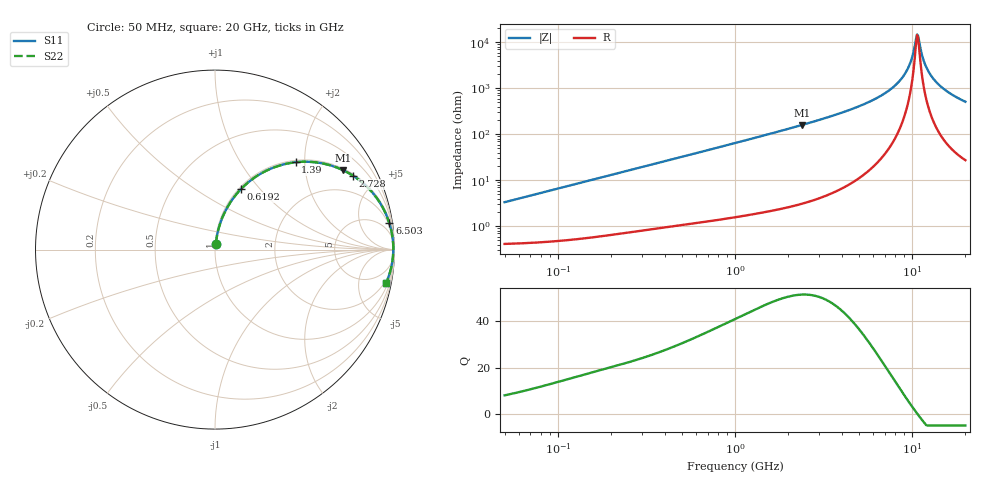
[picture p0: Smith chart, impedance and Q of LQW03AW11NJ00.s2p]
!Murata Part Number: LQW03AW11NJ00
!These Parameters are Measured in Series Mode Connection
!  o--[Z]--o
!Port1  Port2
!  o-------o
!Freq. Start=50[MHz] Stop=20[GHz], 401[Steps]
# Hz S RI R 50
!Freq.(Hz) S11(Real) S11(Imag) S21(Real) S21(Imag) S12(Real) S12(Imag) S22(Real) S22(Imag)
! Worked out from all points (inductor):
!   401 points, 50 MHz to 20 GHz, reference 50 ohm
!   read as one part in series: L = 10.6 nH near 51.52 MHz
!   highest Q = 51.5 at 2.384 GHz (marker M1), where L = 10.6 nH
!   self-resonance near 10.66 GHz
!   S11 on the Smith chart (normalised r, x): 50 MHz: 1.01, +0.07; 619.2 MHz: 1.02, +0.80; 1.39 GHz: 1.04, +1.80; 2.728 GHz: 1.07, +3.70; 6.503 GHz: 2, +13; 20 GHz: 2, -10
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5e7  0.00522 0.0329  0.9948 -0.0329  0.9948 -0.0329  0.00522 0.0329
1.364002e8  0.0133 0.0883  0.9867 -0.0883  0.9867 -0.0883  0.0133 0.0883
3.721004e8  0.0626 0.2243  0.9374 -0.2243  0.9374 -0.2243  0.0626 0.2243
6.192061e8  0.145 0.3375  0.855 -0.3375  0.855 -0.3375  0.145 0.3375
1e9  0.2983 0.4455  0.7017 -0.4455  0.7017 -0.4455  0.2983 0.4455
1.390315e9  0.4493 0.4867  0.5507 -0.4867  0.5507 -0.4867  0.4493 0.4867
2.383959e9  0.7135 0.4425  0.2865 -0.4425  0.2865 -0.4425  0.7135 0.4425
2.728004e9  0.7697 0.4114  0.2303 -0.4114  0.2303 -0.4114  0.7697 0.4114
4.472136e9  0.9163 0.265  0.0837 -0.265  0.0837 -0.265  0.9163 0.265
6.503449e9  0.9713 0.1479  0.0287 -0.1479  0.0287 -0.1479  0.9713 0.1479
7.442007e9  0.9822 0.1071  0.0178 -0.1071  0.0178 -0.1071  0.9822 0.1071
8.516016e9  0.9893 0.0671  0.0107 -0.0671  0.0107 -0.0671  0.9893 0.0671
9.316812e9  0.992 0.0407  0.00796 -0.0407  0.00796 -0.0407  0.992 0.0407
9.892087e9  0.9931 0.0232  0.00693 -0.0232  0.00693 -0.0232  0.9931 0.0232
1.050288e10  0.9935 0.00581  0.00655 -0.00581  0.00655 -0.00581  0.9935 0.00581
1.066139e10  0.9934 0.00146  0.00655 -0.00146  0.00655 -0.00146  0.9934 0.00146
1.098561e10  0.9933 -0.00725  0.00668 0.00725  0.00668 0.00725  0.9933 -0.00725
1.149051e10  0.9928 -0.0203  0.00718 0.0203  0.00718 0.0203  0.9928 -0.0203
1.201863e10  0.992 -0.0334  0.00804 0.0334  0.00804 0.0334  0.992 -0.0334
1.314879e10  0.9891 -0.0596  0.0109 0.0596  0.0109 0.0596  0.9891 -0.0596
1.573793e10  0.9788 -0.1125  0.0212 0.1125  0.0212 0.1125  0.9788 -0.1125
2e10  0.9539 -0.1846  0.0461 0.1846  0.0461 0.1846  0.9539 -0.1846
